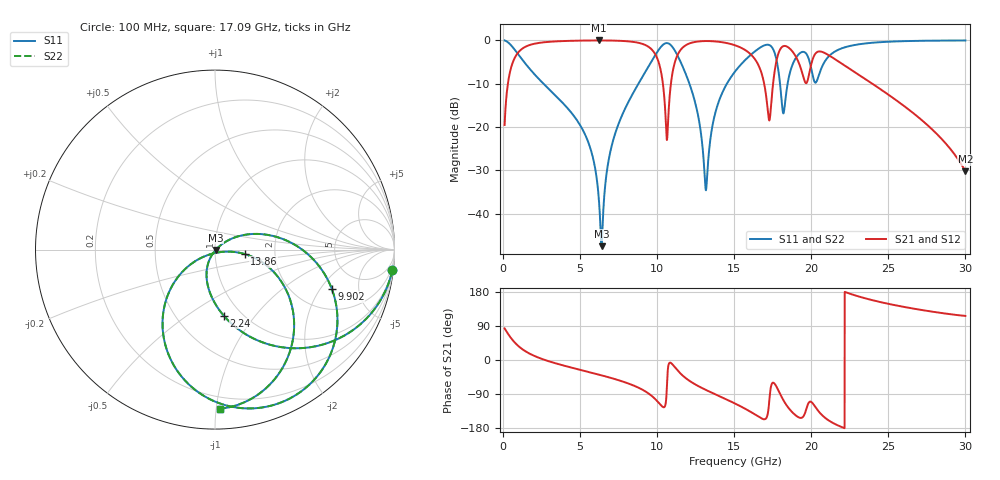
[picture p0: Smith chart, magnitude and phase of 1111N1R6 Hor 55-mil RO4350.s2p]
# GHz S MA R 50
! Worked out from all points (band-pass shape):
!   3201 points, 100 MHz to 30 GHz, reference 50 ohm
!   highest |S21| = -0.04 dB at 6.211 GHz (marker M1); lowest = -30.2 dB at 30 GHz (marker M2)
!   |S21| within 3 dB of the highest: 931.7 MHz to 9.844 GHz (8.913 GHz wide, 165 % of centre); 11.37 GHz to 16.01 GHz (4.636 GHz wide, 33.9 % of centre)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
!   lowest |S11| = -47.5 dB at 6.388 GHz (marker M3), VSWR 1.01, Z = 50.3 - j0.263 ohm
!   |S11| at or under -10 dB: 2.615 GHz to 8.788 GHz (6.173 GHz wide, 108 % of centre); 12.09 GHz to 14.53 GHz (2.439 GHz wide, 18.3 % of centre); 17.97 GHz to 18.46 GHz (494.4 MHz wide, 2.71 % of centre)
!   |S22| runs from -47.5 to 0.0 dB; largest |S21 - S12| = 0
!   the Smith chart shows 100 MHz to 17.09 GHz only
!   S11 on the Smith chart (normalised r, x): 100 MHz: 1, -17; 2.24 GHz: 0.83, -0.71; 9.902 GHz: 3.12, -2.57; 13.86 GHz: 1.39, -0.07; 17.09 GHz: 0.12, -1.03
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0.1  0.9944 -6.7  0.1053 83.3  0.1053 83.3  0.9944 -6.7
0.7260313  0.7911 -42.4  0.6109 47.6  0.6109 47.6  0.7911 -42.4
2.239719  0.3706 -82.5  0.9269 7.2  0.9269 7.2  0.3706 -82.5
5.089563  0.09832 -115.1  0.9915 -26.9  0.9915 -26.9  0.09832 -115.1
6.210813  0.01498 -113.0  0.9952 -38.5  0.9952 -38.5  0.01498 -113.0
6.388344  0.004204 -38.5  0.9951 -40.4  0.9951 -40.4  0.004204 -38.5
7.285344  0.08506 35.5  0.99 -50.7  0.99 -50.7  0.08506 35.5
9.901594  0.6862 -18.5  0.6763 -104.2  0.6763 -104.2  0.6862 -18.5
10.06978  0.763 -27.0  0.5755 -111.5  0.5755 -111.5  0.763 -27.0
10.63975  0.9282 -65.5  0.07088 -60.7  0.07088 -60.7  0.9282 -65.5
11.49003  0.5783 -119.3  0.7618 -34.7  0.7618 -34.7  0.5783 -119.3
13.15322  0.0187 -85.1  0.98 -78.8  0.98 -78.8  0.0187 -85.1
13.86334  0.1663 -8.4  0.9669 -92.3  0.9669 -92.3  0.1663 -8.4
15.05  0.4355 -27.8  0.8756 -114.8  0.8756 -114.8  0.4355 -27.8
17.08694  0.887 -88.1  0.2157 -152.9  0.2157 -152.9  0.887 -88.1
17.67559  0.6657 -129.2  0.5035 -65.7  0.5035 -65.7  0.6657 -129.2
18.1895  0.1432 -98.2  0.856 -106.0  0.856 -106.0  0.1432 -98.2
19.37616  0.7302 -87.1  0.4409 -152.4  0.4409 -152.4  0.7302 -87.1
20.03956  0.4346 -116.5  0.564 -112.0  0.564 -112.0  0.4346 -116.5
21.02066  0.6191 -75.6  0.6902 -156.4  0.6902 -156.4  0.6191 -75.6
25.01978  0.9627 -123.6  0.2345 148.1  0.2345 148.1  0.9627 -123.6
30  0.9946 -157.0  0.03074 116.3  0.03074 116.3  0.9946 -157.0
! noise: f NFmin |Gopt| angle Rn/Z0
0.1  0.001993  0.9204  2.952  0.005532
3.417  0.0121  0.5583  24.42  0.004713
6.743  0.0242  0.5693  42.28  0.008928
10.06  0.1446  0.8757  61.25  0.1864
13.39  0.06467  0.6744  79.95  0.02308
16.7  0.2638  0.8904  96.76  0.2323
20.03  0.5029  0.9296  113.9  0.4739
23.35  0.1901  0.8117  126.3  0.04485
26.67  0.3346  0.8909  141.2  0.07571
30  1.28  0.9713  157.7  0.387
